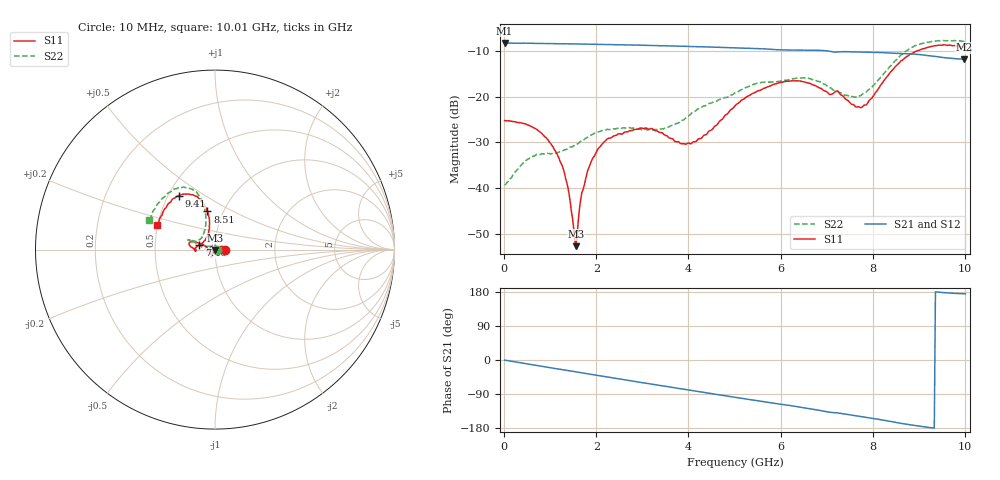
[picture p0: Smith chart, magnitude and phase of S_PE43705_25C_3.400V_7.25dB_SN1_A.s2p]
! Device ID: PE43705
! Serial: 1
! Insertion: A
! Impedance: 50 ohm
! Temp: 25C
! VDD: 3.400V
! Attenuation Step: 7.25dB
#  Hz  S  RI  R  50
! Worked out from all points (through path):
!   401 points, 10 MHz to 10.01 GHz, reference 50 ohm
!   highest |S21| = -8.29 dB at 10 MHz (marker M1); lowest = -11.8 dB at 9.985 GHz (marker M2)
!   group delay of S21, straight-line fit = 52.8 ps
!   lowest |S11| = -52.7 dB at 1.56 GHz (marker M3), VSWR 1.00, Z = 50.1 - j0.204 ohm
!   |S11| at or under -10 dB: start of sweep to 8.968 GHz
!   |S22| runs from -39.3 to -7.7 dB; largest |S21 - S12| = 0.0032
!   S11 on the Smith chart (normalised r, x): 10 MHz: 1.12, -0.00; 7.46 GHz: 0.84, +0.04; 8.51 GHz: 0.84, +0.38; 9.41 GHz: 0.57, +0.39; 10.01 GHz: 0.50, +0.16
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1e7  0.0545 -5.27e-05  0.3848 -0.00187  0.3851 -0.0018  0.0108 0.000329
5.35e8  0.046 0.0158  0.3744 -0.073  0.3745 -0.0728  0.00623 0.0199
1.085e9  0.023 0.0133  0.3505 -0.1413  0.3507 -0.1413  -0.0117 0.0207
1.335e9  0.0111 0.00609  0.3363 -0.1705  0.3364 -0.1703  -0.0212 0.0157
1.51e9  0.00357 -0.000415  0.3242 -0.1902  0.3243 -0.19  -0.0268 0.0109
1.56e9  0.00109 -0.00204  0.3206 -0.1955  0.3209 -0.1955  -0.0284 0.00932
1.685e9  -0.00388 -0.00798  0.3114 -0.2086  0.3115 -0.2086  -0.0325 0.0052
1.885e9  -0.0111 -0.0157  0.2952 -0.2288  0.2953 -0.2284  -0.0379 -0.000764
2.21e9  -0.0168 -0.0286  0.2661 -0.2587  0.2661 -0.2587  -0.0422 -0.00936
2.935e9  -0.0202 -0.04  0.1904 -0.3109  0.1908 -0.311  -0.0427 -0.0109
3.36e9  -0.0179 -0.0367  0.1422 -0.3304  0.1426 -0.3302  -0.0423 -0.00914
4.085e9  -0.0299 -0.01  0.0573 -0.3469  0.0576 -0.3469  -0.0665 0.00899
5.01e9  -0.0727 0.031  -0.0498 -0.3364  -0.0492 -0.3365  -0.1038 0.0355
5.96e9  -0.1338 0.0441  -0.1424 -0.2919  -0.1415 -0.2919  -0.1361 0.0537
6.685e9  -0.1341 0.0155  -0.2041 -0.2476  -0.2039 -0.2474  -0.1442 0.0525
7.46e9  -0.0868 0.0255  -0.2496 -0.182  -0.2487 -0.1824  -0.085 0.0571
7.81e9  -0.0517 0.0616  -0.2661 -0.1509  -0.266 -0.1512  -0.0656 0.0868
8.36e9  -0.032 0.1755  -0.2843 -0.0947  -0.2835 -0.096  -0.0537 0.2026
8.51e9  -0.0424 0.2128  -0.2859 -0.0767  -0.2848 -0.0789  -0.0627 0.2432
9.41e9  -0.2025 0.3012  -0.2718 0.00343  -0.2713 0.00369  -0.2311 0.3356
9.985e9  -0.3138 0.1458  -0.2547 0.0231  -0.2553 0.0228  -0.3584 0.1774
1.001e10  -0.3209 0.1368  -0.2555 0.0237  -0.256 0.0228  -0.3663 0.1661
